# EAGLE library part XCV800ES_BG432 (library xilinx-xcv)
xcv800es_bg432 edit this description Auto generated by make-symbol-device-package-bsdl.ulp Rev. 26 Source: xcv800es_bg432.bsd
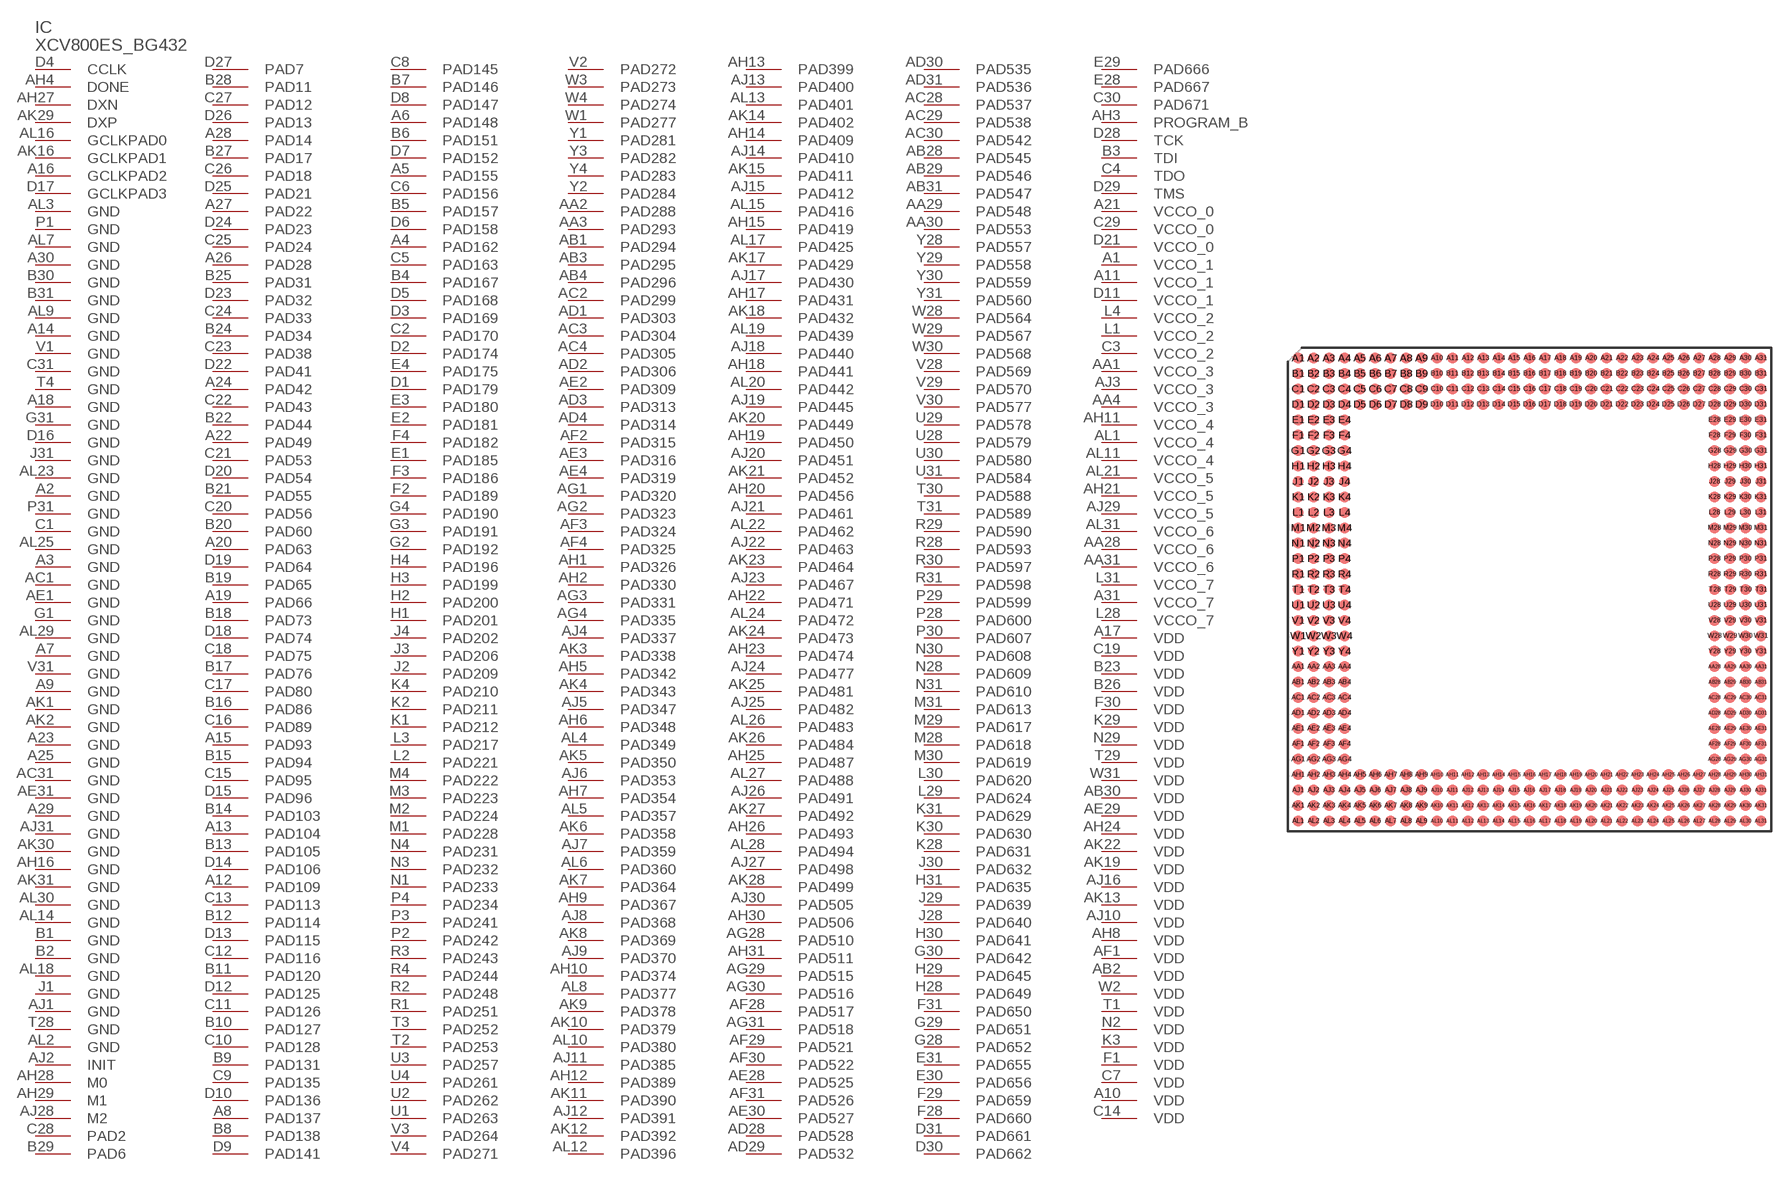
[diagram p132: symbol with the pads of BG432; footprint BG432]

Designator prefix IC

## XCV800ES_BG432 (OC_FARNELL: unknown; OC_NEWARK: unknown)  [BG432]
A1  VCCO_1  pwr
A2  GND  pwr
A3  GND  pwr
A4  PAD162
A5  PAD155
A6  PAD148
A7  GND  pwr
A8  PAD137
A9  GND  pwr
A10  VDD  pwr
A11  VCCO_1  pwr
A12  PAD109
A13  PAD104
A14  GND  pwr
A15  PAD93
A16  GCLKPAD2  in
A17  VDD  pwr
A18  GND  pwr
A19  PAD66
A20  PAD63
A21  VCCO_0  pwr
A22  PAD49
A23  GND  pwr
A24  PAD42
A25  GND  pwr
A26  PAD28
A27  PAD22
A28  PAD14
A29  GND  pwr
A30  GND  pwr
A31  VCCO_7  pwr
AA1  VCCO_3  pwr
AA2  PAD288
AA3  PAD293
AA4  VCCO_3  pwr
AA28  VCCO_6  pwr
AA29  PAD548
AA30  PAD553
AA31  VCCO_6  pwr
AB1  PAD294
AB2  VDD  pwr
AB3  PAD295
AB4  PAD296
AB28  PAD545
AB29  PAD546
AB30  VDD  pwr
AB31  PAD547
AC1  GND  pwr
AC2  PAD299
AC3  PAD304
AC4  PAD305
AC28  PAD537
AC29  PAD538
AC30  PAD542
AC31  GND  pwr
AD1  PAD303
AD2  PAD306
AD3  PAD313
AD4  PAD314
AD28  PAD528
AD29  PAD532
AD30  PAD535
AD31  PAD536
AE1  GND  pwr
AE2  PAD309
AE3  PAD316
AE4  PAD319
AE28  PAD525
AE29  VDD  pwr
AE30  PAD527
AE31  GND  pwr
AF1  VDD  pwr
AF2  PAD315
AF3  PAD324
AF4  PAD325
AF28  PAD517
AF29  PAD521
AF30  PAD522
AF31  PAD526
AG1  PAD320
AG2  PAD323
AG3  PAD331
AG4  PAD335
AG28  PAD510
AG29  PAD515
AG30  PAD516
AG31  PAD518
AH1  PAD326
AH2  PAD330
AH3  PROGRAM_B  in
AH4  DONE
AH5  PAD342
AH6  PAD348
AH7  PAD354
AH8  VDD  pwr
AH9  PAD367
AH10  PAD374
AH11  VCCO_4  pwr
AH12  PAD389
AH13  PAD399
AH14  PAD409
AH15  PAD419
AH16  GND  pwr
AH17  PAD431
AH18  PAD441
AH19  PAD450
AH20  PAD456
AH21  VCCO_5  pwr
AH22  PAD471
AH23  PAD474
AH24  VDD  pwr
AH25  PAD487
AH26  PAD493
AH27  DXN  pas
AH28  M0  in
AH29  M1  in
AH30  PAD506
AH31  PAD511
AJ1  GND  pwr
AJ2  INIT
AJ3  VCCO_3  pwr
AJ4  PAD337
AJ5  PAD347
AJ6  PAD353
AJ7  PAD359
AJ8  PAD368
AJ9  PAD370
AJ10  VDD  pwr
AJ11  PAD385
AJ12  PAD391
AJ13  PAD400
AJ14  PAD410
AJ15  PAD412
AJ16  VDD  pwr
AJ17  PAD430
AJ18  PAD440
AJ19  PAD445
AJ20  PAD451
AJ21  PAD461
AJ22  PAD463
AJ23  PAD467
AJ24  PAD477
AJ25  PAD482
AJ26  PAD491
AJ27  PAD498
AJ28  M2  in
AJ29  VCCO_5  pwr
AJ30  PAD505
AJ31  GND  pwr
AK1  GND  pwr
AK2  GND  pwr
AK3  PAD338
AK4  PAD343
AK5  PAD350
AK6  PAD358
AK7  PAD364
AK8  PAD369
AK9  PAD378
AK10  PAD379
AK11  PAD390
AK12  PAD392
AK13  VDD  pwr
AK14  PAD402
AK15  PAD411
AK16  GCLKPAD1  in
AK17  PAD429
AK18  PAD432
AK19  VDD  pwr
AK20  PAD449
AK21  PAD452
AK22  VDD  pwr
AK23  PAD464
AK24  PAD473
AK25  PAD481
AK26  PAD484
AK27  PAD492
AK28  PAD499
AK29  DXP  pas
AK30  GND  pwr
AK31  GND  pwr
AL1  VCCO_4  pwr
AL2  GND  pwr
AL3  GND  pwr
AL4  PAD349
AL5  PAD357
AL6  PAD360
AL7  GND  pwr
AL8  PAD377
AL9  GND  pwr
AL10  PAD380
AL11  VCCO_4  pwr
AL12  PAD396
AL13  PAD401
AL14  GND  pwr
AL15  PAD416
AL16  GCLKPAD0  in
AL17  PAD425
AL18  GND  pwr
AL19  PAD439
AL20  PAD442
AL21  VCCO_5  pwr
AL22  PAD462
AL23  GND  pwr
AL24  PAD472
AL25  GND  pwr
AL26  PAD483
AL27  PAD488
AL28  PAD494
AL29  GND  pwr
AL30  GND  pwr
AL31  VCCO_6  pwr
B1  GND  pwr
B2  GND  pwr
B3  TDI  in
B4  PAD167
B5  PAD157
B6  PAD151
B7  PAD146
B8  PAD138
B9  PAD131
B10  PAD127
B11  PAD120
B12  PAD114
B13  PAD105
B14  PAD103
B15  PAD94
B16  PAD86
B17  PAD76
B18  PAD73
B19  PAD65
B20  PAD60
B21  PAD55
B22  PAD44
B23  VDD  pwr
B24  PAD34
B25  PAD31
B26  VDD  pwr
B27  PAD17
B28  PAD11
B29  PAD6
B30  GND  pwr
B31  GND  pwr
C1  GND  pwr
C2  PAD170
C3  VCCO_2  pwr
C4  TDO  out
C5  PAD163
C6  PAD156
C7  VDD  pwr
C8  PAD145
C9  PAD135
C10  PAD128
C11  PAD126
C12  PAD116
C13  PAD113
C14  VDD  pwr
C15  PAD95
C16  PAD89
C17  PAD80
C18  PAD75
C19  VDD  pwr
C20  PAD56
C21  PAD53
C22  PAD43
C23  PAD38
C24  PAD33
C25  PAD24
C26  PAD18
C27  PAD12
C28  PAD2
C29  VCCO_0  pwr
C30  PAD671
C31  GND  pwr
D1  PAD179
D2  PAD174
D3  PAD169
D4  CCLK
D5  PAD168
D6  PAD158
D7  PAD152
D8  PAD147
D9  PAD141
D10  PAD136
D11  VCCO_1  pwr
D12  PAD125
D13  PAD115
D14  PAD106
D15  PAD96
D16  GND  pwr
D17  GCLKPAD3  in
D18  PAD74
D19  PAD64
D20  PAD54
D21  VCCO_0  pwr
D22  PAD41
D23  PAD32
D24  PAD23
D25  PAD21
D26  PAD13
D27  PAD7
D28  TCK  in
D29  TMS  in
D30  PAD662
D31  PAD661
E1  PAD185
E2  PAD181
E3  PAD180
E4  PAD175
E28  PAD667
E29  PAD666
E30  PAD656
E31  PAD655
F1  VDD  pwr
F2  PAD189
F3  PAD186
F4  PAD182
F28  PAD660
F29  PAD659
F30  VDD  pwr
F31  PAD650
G1  GND  pwr
G2  PAD192
G3  PAD191
G4  PAD190
G28  PAD652
G29  PAD651
G30  PAD642
G31  GND  pwr
H1  PAD201
H2  PAD200
H3  PAD199
H4  PAD196
H28  PAD649
H29  PAD645
H30  PAD641
H31  PAD635
J1  GND  pwr
J2  PAD209
J3  PAD206
J4  PAD202
J28  PAD640
J29  PAD639
J30  PAD632
J31  GND  pwr
K1  PAD212
K2  PAD211
K3  VDD  pwr
K4  PAD210
K28  PAD631
K29  VDD  pwr
K30  PAD630
K31  PAD629
L1  VCCO_2  pwr
L2  PAD221
L3  PAD217
L4  VCCO_2  pwr
L28  VCCO_7  pwr
L29  PAD624
L30  PAD620
L31  VCCO_7  pwr
M1  PAD228
M2  PAD224
M3  PAD223
M4  PAD222
M28  PAD618
M29  PAD617
M30  PAD619
M31  PAD613
N1  PAD233
N2  VDD  pwr
N3  PAD232
N4  PAD231
N28  PAD609
N29  VDD  pwr
N30  PAD608
N31  PAD610
P1  GND  pwr
P2  PAD242
P3  PAD241
P4  PAD234
P28  PAD600
P29  PAD599
P30  PAD607
P31  GND  pwr
R1  PAD251
R2  PAD248
R3  PAD243
R4  PAD244
R28  PAD593
R29  PAD590
R30  PAD597
R31  PAD598
T1  VDD  pwr
T2  PAD253
T3  PAD252
T4  GND  pwr
T28  GND  pwr
T29  VDD  pwr
T30  PAD588
T31  PAD589
U1  PAD263
U2  PAD262
U3  PAD257
U4  PAD261
U28  PAD579
U29  PAD578
U30  PAD580
U31  PAD584
V1  GND  pwr
V2  PAD272
V3  PAD264
V4  PAD271
V28  PAD569
V29  PAD570
V30  PAD577
V31  GND  pwr
W1  PAD277
W2  VDD  pwr
W3  PAD273
W4  PAD274
W28  PAD564
W29  PAD567
W30  PAD568
W31  VDD  pwr
Y1  PAD281
Y2  PAD284
Y3  PAD282
Y4  PAD283
Y28  PAD557
Y29  PAD558
Y30  PAD559
Y31  PAD560

## Footprint BG432 (pad centres in mm)
xcv300_bg432 edit this description Auto generated by make-symbol-device-package-bsdl.ulp Rev. 26 Source: xcv300_bg432.bsd
smd 0.9 x 0.9: A1 -19.05,19.05; A2 -17.78,19.05; A3 -16.51,19.05; A4 -15.24,19.05; A5 -13.97,19.05; A6 -12.7,19.05; A7 -11.43,19.05; A8 -10.16,19.05; A9 -8.89,19.05; A10 -7.62,19.05; A11 -6.35,19.05; A12 -5.08,19.05; A13 -3.81,19.05; A14 -2.54,19.05; A15 -1.27,19.05; A16 0,19.05; A17 1.27,19.05; A18 2.54,19.05; A19 3.81,19.05; A20 5.08,19.05; A21 6.35,19.05; A22 7.62,19.05; A23 8.89,19.05; A24 10.16,19.05; A25 11.43,19.05; A26 12.7,19.05; A27 13.97,19.05; A28 15.24,19.05; A29 16.51,19.05; A30 17.78,19.05; A31 19.05,19.05; AA1 -19.05,-6.35; AA2 -17.78,-6.35; AA3 -16.51,-6.35; AA4 -15.24,-6.35; AA28 15.24,-6.35; AA29 16.51,-6.35; AA30 17.78,-6.35; AA31 19.05,-6.35; AB1 -19.05,-7.62; AB2 -17.78,-7.62; AB3 -16.51,-7.62; AB4 -15.24,-7.62; AB28 15.24,-7.62; AB29 16.51,-7.62; AB30 17.78,-7.62; AB31 19.05,-7.62; AC1 -19.05,-8.89; AC2 -17.78,-8.89; AC3 -16.51,-8.89; AC4 -15.24,-8.89; AC28 15.24,-8.89; AC29 16.51,-8.89; AC30 17.78,-8.89; AC31 19.05,-8.89; AD1 -19.05,-10.16; AD2 -17.78,-10.16; AD3 -16.51,-10.16; AD4 -15.24,-10.16; AD28 15.24,-10.16; AD29 16.51,-10.16; AD30 17.78,-10.16; AD31 19.05,-10.16; AE1 -19.05,-11.43; AE2 -17.78,-11.43; AE3 -16.51,-11.43; AE4 -15.24,-11.43; AE28 15.24,-11.43; AE29 16.51,-11.43; AE30 17.78,-11.43; AE31 19.05,-11.43; AF1 -19.05,-12.7; AF2 -17.78,-12.7; AF3 -16.51,-12.7; AF4 -15.24,-12.7; AF28 15.24,-12.7; AF29 16.51,-12.7; AF30 17.78,-12.7; AF31 19.05,-12.7; AG1 -19.05,-13.97; AG2 -17.78,-13.97; AG3 -16.51,-13.97; AG4 -15.24,-13.97; AG28 15.24,-13.97; AG29 16.51,-13.97; AG30 17.78,-13.97; AG31 19.05,-13.97; AH1 -19.05,-15.24; AH2 -17.78,-15.24; AH3 -16.51,-15.24; AH4 -15.24,-15.24; AH5 -13.97,-15.24; AH6 -12.7,-15.24; AH7 -11.43,-15.24; AH8 -10.16,-15.24; AH9 -8.89,-15.24; AH10 -7.62,-15.24; AH11 -6.35,-15.24; AH12 -5.08,-15.24; AH13 -3.81,-15.24; AH14 -2.54,-15.24; AH15 -1.27,-15.24; AH16 0,-15.24; AH17 1.27,-15.24; AH18 2.54,-15.24; AH19 3.81,-15.24; AH20 5.08,-15.24; AH21 6.35,-15.24; AH22 7.62,-15.24; AH23 8.89,-15.24; AH24 10.16,-15.24; AH25 11.43,-15.24; AH26 12.7,-15.24; AH27 13.97,-15.24; AH28 15.24,-15.24; AH29 16.51,-15.24; AH30 17.78,-15.24; AH31 19.05,-15.24; AJ1 -19.05,-16.51; AJ2 -17.78,-16.51; AJ3 -16.51,-16.51; AJ4 -15.24,-16.51; AJ5 -13.97,-16.51; AJ6 -12.7,-16.51; AJ7 -11.43,-16.51; AJ8 -10.16,-16.51; AJ9 -8.89,-16.51; AJ10 -7.62,-16.51; AJ11 -6.35,-16.51; AJ12 -5.08,-16.51; AJ13 -3.81,-16.51; AJ14 -2.54,-16.51; AJ15 -1.27,-16.51; AJ16 0,-16.51; AJ17 1.27,-16.51; AJ18 2.54,-16.51; AJ19 3.81,-16.51; AJ20 5.08,-16.51; AJ21 6.35,-16.51; AJ22 7.62,-16.51; AJ23 8.89,-16.51; AJ24 10.16,-16.51; AJ25 11.43,-16.51; AJ26 12.7,-16.51; AJ27 13.97,-16.51; AJ28 15.24,-16.51; AJ29 16.51,-16.51; AJ30 17.78,-16.51; AJ31 19.05,-16.51; AK1 -19.05,-17.78; AK2 -17.78,-17.78; AK3 -16.51,-17.78; AK4 -15.24,-17.78; AK5 -13.97,-17.78; AK6 -12.7,-17.78; AK7 -11.43,-17.78; AK8 -10.16,-17.78; AK9 -8.89,-17.78; AK10 -7.62,-17.78; AK11 -6.35,-17.78; AK12 -5.08,-17.78; AK13 -3.81,-17.78; AK14 -2.54,-17.78; AK15 -1.27,-17.78; AK16 0,-17.78; AK17 1.27,-17.78; AK18 2.54,-17.78; AK19 3.81,-17.78; AK20 5.08,-17.78; AK21 6.35,-17.78; AK22 7.62,-17.78; AK23 8.89,-17.78; AK24 10.16,-17.78; AK25 11.43,-17.78; AK26 12.7,-17.78; AK27 13.97,-17.78; AK28 15.24,-17.78; AK29 16.51,-17.78; AK30 17.78,-17.78; AK31 19.05,-17.78; AL1 -19.05,-19.05; AL2 -17.78,-19.05; AL3 -16.51,-19.05; AL4 -15.24,-19.05; AL5 -13.97,-19.05; AL6 -12.7,-19.05; AL7 -11.43,-19.05; AL8 -10.16,-19.05; AL9 -8.89,-19.05; AL10 -7.62,-19.05; AL11 -6.35,-19.05; AL12 -5.08,-19.05; AL13 -3.81,-19.05; AL14 -2.54,-19.05; AL15 -1.27,-19.05; AL16 0,-19.05; AL17 1.27,-19.05; AL18 2.54,-19.05; AL19 3.81,-19.05; AL20 5.08,-19.05; AL21 6.35,-19.05; AL22 7.62,-19.05; AL23 8.89,-19.05; AL24 10.16,-19.05; AL25 11.43,-19.05; AL26 12.7,-19.05; AL27 13.97,-19.05; AL28 15.24,-19.05; AL29 16.51,-19.05; AL30 17.78,-19.05; AL31 19.05,-19.05; B1 -19.05,17.78; B2 -17.78,17.78; B3 -16.51,17.78; B4 -15.24,17.78; B5 -13.97,17.78; B6 -12.7,17.78; B7 -11.43,17.78; B8 -10.16,17.78; B9 -8.89,17.78; B10 -7.62,17.78; B11 -6.35,17.78; B12 -5.08,17.78; B13 -3.81,17.78; B14 -2.54,17.78; B15 -1.27,17.78; B16 0,17.78; B17 1.27,17.78; B18 2.54,17.78; B19 3.81,17.78; B20 5.08,17.78; B21 6.35,17.78; B22 7.62,17.78; B23 8.89,17.78; B24 10.16,17.78; B25 11.43,17.78; B26 12.7,17.78; B27 13.97,17.78; B28 15.24,17.78; B29 16.51,17.78; B30 17.78,17.78; B31 19.05,17.78; C1 -19.05,16.51; C2 -17.78,16.51; C3 -16.51,16.51; C4 -15.24,16.51; C5 -13.97,16.51; C6 -12.7,16.51; C7 -11.43,16.51; C8 -10.16,16.51; C9 -8.89,16.51; C10 -7.62,16.51; C11 -6.35,16.51; C12 -5.08,16.51; C13 -3.81,16.51; C14 -2.54,16.51; C15 -1.27,16.51; C16 0,16.51; C17 1.27,16.51; C18 2.54,16.51; C19 3.81,16.51; C20 5.08,16.51; C21 6.35,16.51; C22 7.62,16.51; C23 8.89,16.51; C24 10.16,16.51; C25 11.43,16.51; C26 12.7,16.51; C27 13.97,16.51; C28 15.24,16.51; C29 16.51,16.51; C30 17.78,16.51; C31 19.05,16.51; D1 -19.05,15.24; D2 -17.78,15.24; D3 -16.51,15.24; D4 -15.24,15.24; D5 -13.97,15.24; D6 -12.7,15.24; D7 -11.43,15.24; D8 -10.16,15.24; D9 -8.89,15.24; D10 -7.62,15.24; D11 -6.35,15.24; D12 -5.08,15.24; D13 -3.81,15.24; D14 -2.54,15.24; D15 -1.27,15.24; D16 0,15.24; D17 1.27,15.24; D18 2.54,15.24; D19 3.81,15.24; D20 5.08,15.24; D21 6.35,15.24; D22 7.62,15.24; D23 8.89,15.24; D24 10.16,15.24; D25 11.43,15.24; D26 12.7,15.24; D27 13.97,15.24; D28 15.24,15.24; D29 16.51,15.24; D30 17.78,15.24; D31 19.05,15.24; E1 -19.05,13.97; E2 -17.78,13.97; E3 -16.51,13.97; E4 -15.24,13.97; E28 15.24,13.97; E29 16.51,13.97; E30 17.78,13.97; E31 19.05,13.97; F1 -19.05,12.7; F2 -17.78,12.7; F3 -16.51,12.7; F4 -15.24,12.7; F28 15.24,12.7; F29 16.51,12.7; F30 17.78,12.7; F31 19.05,12.7; G1 -19.05,11.43; G2 -17.78,11.43; G3 -16.51,11.43; G4 -15.24,11.43; G28 15.24,11.43; G29 16.51,11.43; G30 17.78,11.43; G31 19.05,11.43; H1 -19.05,10.16; H2 -17.78,10.16; H3 -16.51,10.16; H4 -15.24,10.16; H28 15.24,10.16; H29 16.51,10.16; H30 17.78,10.16; H31 19.05,10.16; J1 -19.05,8.89; J2 -17.78,8.89; J3 -16.51,8.89; J4 -15.24,8.89; J28 15.24,8.89; J29 16.51,8.89; J30 17.78,8.89; J31 19.05,8.89; K1 -19.05,7.62; K2 -17.78,7.62; K3 -16.51,7.62; K4 -15.24,7.62; K28 15.24,7.62; K29 16.51,7.62; K30 17.78,7.62; K31 19.05,7.62; L1 -19.05,6.35; L2 -17.78,6.35; L3 -16.51,6.35; L4 -15.24,6.35; L28 15.24,6.35; L29 16.51,6.35; L30 17.78,6.35; L31 19.05,6.35; M1 -19.05,5.08; M2 -17.78,5.08; M3 -16.51,5.08; M4 -15.24,5.08; M28 15.24,5.08; M29 16.51,5.08; M30 17.78,5.08; M31 19.05,5.08; N1 -19.05,3.81; N2 -17.78,3.81; N3 -16.51,3.81; N4 -15.24,3.81; N28 15.24,3.81; N29 16.51,3.81; N30 17.78,3.81; N31 19.05,3.81; P1 -19.05,2.54; P2 -17.78,2.54; P3 -16.51,2.54; P4 -15.24,2.54; P28 15.24,2.54; P29 16.51,2.54; P30 17.78,2.54; P31 19.05,2.54; R1 -19.05,1.27; R2 -17.78,1.27; R3 -16.51,1.27; R4 -15.24,1.27; R28 15.24,1.27; R29 16.51,1.27; R30 17.78,1.27; R31 19.05,1.27; T1 -19.05,0; T2 -17.78,0; T3 -16.51,0; T4 -15.24,0; T28 15.24,0; T29 16.51,0; T30 17.78,0; T31 19.05,0; U1 -19.05,-1.27; U2 -17.78,-1.27; U3 -16.51,-1.27; U4 -15.24,-1.27; U28 15.24,-1.27; U29 16.51,-1.27; U30 17.78,-1.27; U31 19.05,-1.27; V1 -19.05,-2.54; V2 -17.78,-2.54; V3 -16.51,-2.54; V4 -15.24,-2.54; V28 15.24,-2.54; V29 16.51,-2.54; V30 17.78,-2.54; V31 19.05,-2.54; W1 -19.05,-3.81; W2 -17.78,-3.81; W3 -16.51,-3.81; W4 -15.24,-3.81; W28 15.24,-3.81; W29 16.51,-3.81; W30 17.78,-3.81; W31 19.05,-3.81; Y1 -19.05,-5.08; Y2 -17.78,-5.08; Y3 -16.51,-5.08; Y4 -15.24,-5.08; Y28 15.24,-5.08; Y29 16.51,-5.08; Y30 17.78,-5.08; Y31 19.05,-5.08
